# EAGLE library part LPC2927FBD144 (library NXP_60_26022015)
Short The LPC2926/2927/2929 combine an ARM968E-S CPU core with two integrated TCM blocks operating at frequencies of up to 125 MHz, Full-speed USB 2.0 OTG and device controller, CAN and LIN, 56 kB SRAM, up to 768 kB flash memory, external memory interface, three 10-bit ADCs, and multiple serial and parallel interfaces in a single chip targeted at consumer, industrial and communication markets. To optimize system power consumption, the LPC2926/2927/2929 has a very flexible Clock Generation Unit (CGU) that provides dynamic clock gating and scaling. AAL Eindhoven MK
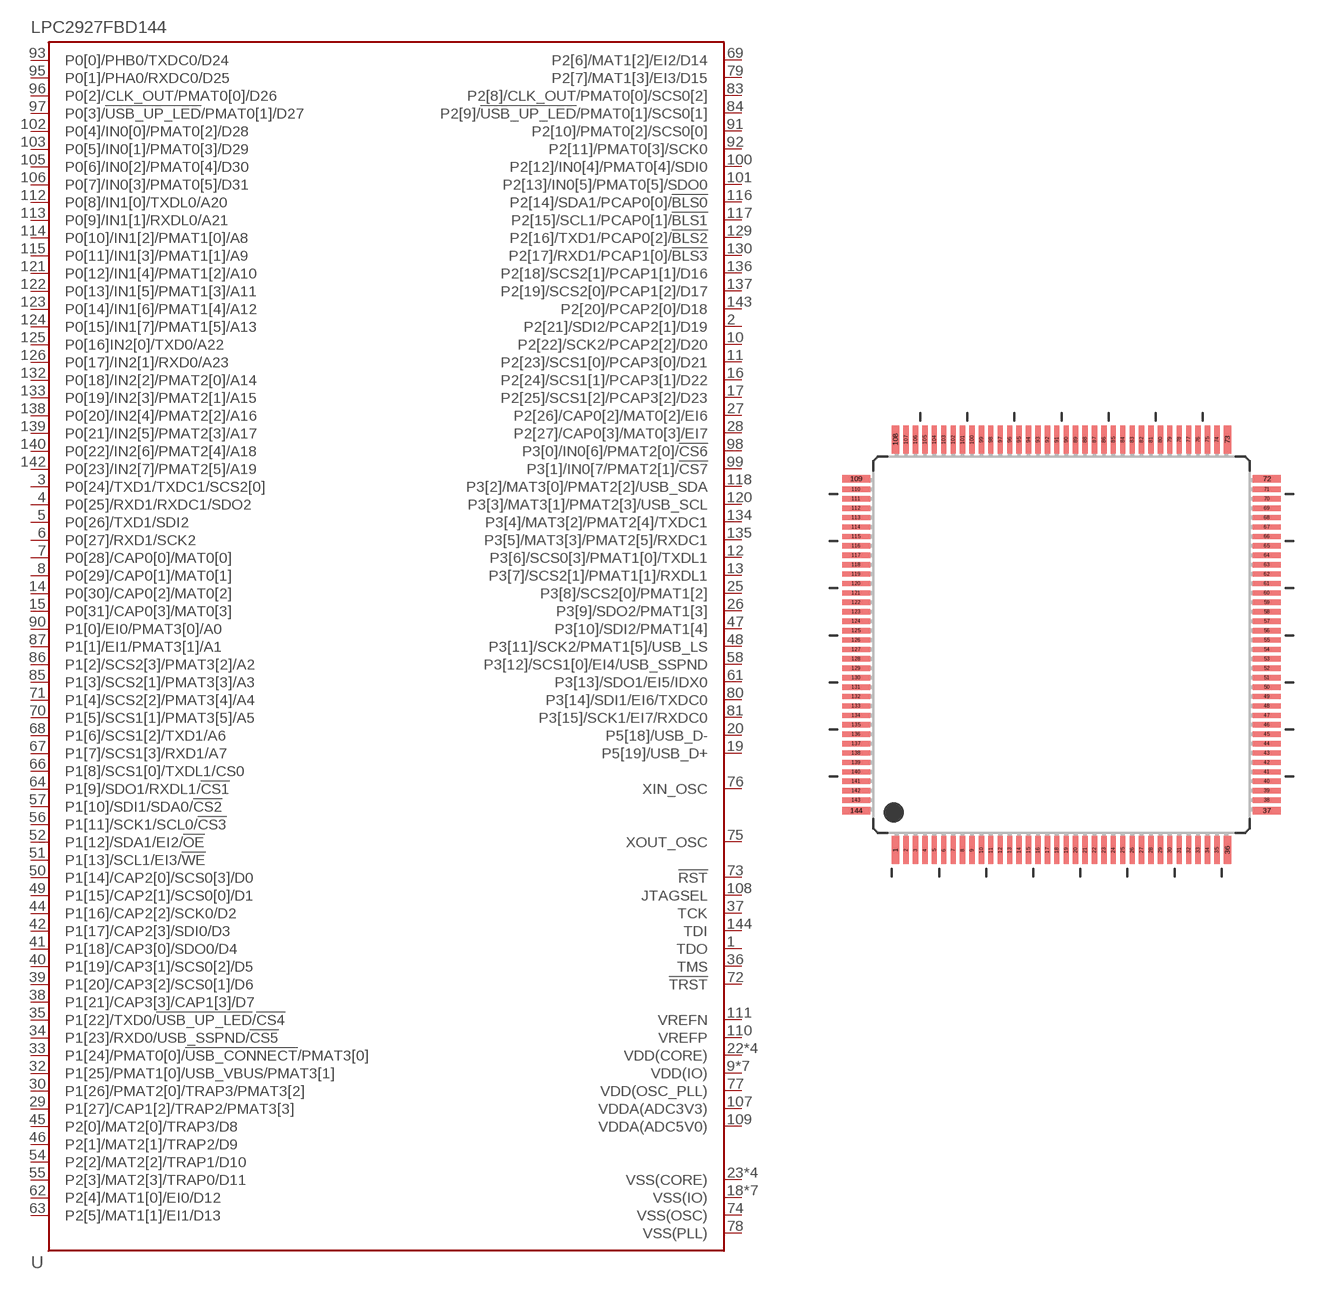
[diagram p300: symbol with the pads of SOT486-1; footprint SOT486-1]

Designator prefix U

## LPC2927FBD144 (FLASH: 512kB; SRAM: 56kB + 2 × 32kB TCM)  [SOT486-1]
1  TDO
2  P2[21]/SDI2/PCAP2[1]/D19
3  P0[24]/TXD1/TXDC1/SCS2[0]
4  P0[25]/RXD1/RXDC1/SDO2
5  P0[26]/TXD1/SDI2
6  P0[27]/RXD1/SCK2
7  P0[28]/CAP0[0]/MAT0[0]
8  P0[29]/CAP0[1]/MAT0[1]
9  VDD(IO)
10  P2[22]/SCK2/PCAP2[2]/D20
11  P2[23]/SCS1[0]/PCAP3[0]/D21
12  P3[6]/SCS0[3]/PMAT1[0]/TXDL1
13  P3[7]/SCS2[1]/PMAT1[1]/RXDL1
14  P0[30]/CAP0[2]/MAT0[2]
15  P0[31]/CAP0[3]/MAT0[3]
16  P2[24]/SCS1[1]/PCAP3[1]/D22
17  P2[25]/SCS1[2]/PCAP3[2]/D23
18  VSS(IO)
19  P5[19]/USB_D+
20  P5[18]/USB_D-
21  VDD(IO)
22  VDD(CORE)
23  VSS(CORE)
24  VSS(IO)
25  P3[8]/SCS2[0]/PMAT1[2]
26  P3[9]/SDO2/PMAT1[3]
27  P2[26]/CAP0[2]/MAT0[2]/EI6
28  P2[27]/CAP0[3]/MAT0[3]/EI7
29  P1[27]/CAP1[2]/TRAP2/PMAT3[3]
30  P1[26]/PMAT2[0]/TRAP3/PMAT3[2]
31  VDD(IO)
32  P1[25]/PMAT1[0]/USB_VBUS/PMAT3[1]
33  P1[24]/PMAT0[0]/!USB_CONNECT!/PMAT3[0]
34  P1[23]/RXD0/USB_SSPND/!CS5!
35  P1[22]/TXD0/!USB_UP_LED!/!CS4!
36  TMS
37  TCK
38  P1[21]/CAP3[3]/CAP1[3]/D7
39  P1[20]/CAP3[2]/SCS0[1]/D6
40  P1[19]/CAP3[1]/SCS0[2]/D5
41  P1[18]/CAP3[0]/SDO0/D4
42  P1[17]/CAP2[3]/SDI0/D3
43  VSS(IO)
44  P1[16]/CAP2[2]/SCK0/D2
45  P2[0]/MAT2[0]/TRAP3/D8
46  P2[1]/MAT2[1]/TRAP2/D9
47  P3[10]/SDI2/PMAT1[4]
48  P3[11]/SCK2/PMAT1[5]/USB_LS
49  P1[15]/CAP2[1]/SCS0[0]/D1
50  P1[14]/CAP2[0]/SCS0[3]/D0
51  P1[13]/SCL1/EI3/!WE!
52  P1[12]/SDA1/EI2/!OE!
53  VDD(IO)
54  P2[2]/MAT2[2]/TRAP1/D10
55  P2[3]/MAT2[3]/TRAP0/D11
56  P1[11]/SCK1/SCL0/!CS3!
57  P1[10]/SDI1/SDA0/!CS2!
58  P3[12]/SCS1[0]/EI4/USB_SSPND
59  VSS(CORE)
60  VDD(CORE)
61  P3[13]/SDO1/EI5/IDX0
62  P2[4]/MAT1[0]/EI0/D12
63  P2[5]/MAT1[1]/EI1/D13
64  P1[9]/SDO1/RXDL1/!CS1!
65  VSS(IO)
66  P1[8]/SCS1[0]/TXDL1/CS0
67  P1[7]/SCS1[3]/RXD1/A7
68  P1[6]/SCS1[2]/TXD1/A6
69  P2[6]/MAT1[2]/EI2/D14
70  P1[5]/SCS1[1]/PMAT3[5]/A5
71  P1[4]/SCS2[2]/PMAT3[4]/A4
72  !TRST!
73  !RST!
74  VSS(OSC)
75  XOUT_OSC
76  XIN_OSC
77  VDD(OSC_PLL)
78  VSS(PLL)
79  P2[7]/MAT1[3]/EI3/D15
80  P3[14]/SDI1/EI6/TXDC0
81  P3[15]/SCK1/EI7/RXDC0
82  VDD(IO)
83  P2[8]/CLK_OUT/PMAT0[0]/SCS0[2]
84  P2[9]/!USB_UP_LED!/PMAT0[1]/SCS0[1]
85  P1[3]/SCS2[1]/PMAT3[3]/A3
86  P1[2]/SCS2[3]/PMAT3[2]/A2
87  P1[1]/EI1/PMAT3[1]/A1
88  VSS(CORE)
89  VDD(CORE)
90  P1[0]/EI0/PMAT3[0]/A0
91  P2[10]/PMAT0[2]/SCS0[0]
92  P2[11]/PMAT0[3]/SCK0
93  P0[0]/PHB0/TXDC0/D24
94  VSS(IO)
95  P0[1]/PHA0/RXDC0/D25
96  P0[2]/CLK_OUT/PMAT0[0]/D26
97  P0[3]/!USB_UP_LED!/PMAT0[1]/D27
98  P3[0]/IN0[6]/PMAT2[0]/!CS6!
99  P3[1]/IN0[7/PMAT2[1]/!CS7!
100  P2[12]/IN0[4]/PMAT0[4]/SDI0
101  P2[13]/IN0[5]/PMAT0[5]/SDO0
102  P0[4]/IN0[0]/PMAT0[2]/D28
103  P0[5]/IN0[1]/PMAT0[3]/D29
104  VDD(IO)
105  P0[6]/IN0[2]/PMAT0[4]/D30
106  P0[7]/IN0[3]/PMAT0[5]/D31
107  VDDA(ADC3V3)
108  JTAGSEL
109  VDDA(ADC5V0)
110  VREFP
111  VREFN
112  P0[8]/IN1[0]/TXDL0/A20
113  P0[9]/IN1[1]/RXDL0/A21
114  P0[10]/IN1[2]/PMAT1[0]/A8
115  P0[11]/IN1[3]/PMAT1[1]/A9
116  P2[14]/SDA1/PCAP0[0]/!BLS0!
117  P2[15]/SCL1/PCAP0[1]/!BLS1!
118  P3[2]/MAT3[0]/PMAT2[2]/USB_SDA
119  VSS(IO)
120  P3[3]/MAT3[1]/PMAT2[3]/USB_SCL
121  P0[12]/IN1[4]/PMAT1[2]/A10
122  P0[13]/IN1[5]/PMAT1[3]/A11
123  P0[14]/IN1[6]/PMAT1[4]/A12
124  P0[15]/IN1[7]/PMAT1[5]/A13
125  P0[16]IN2[0]/TXD0/A22
126  P0[17]/IN2[1]/RXD0/A23
127  VDD(CORE)
128  VSS(CORE)
129  P2[16]/TXD1/PCAP0[2]/!BLS2!
130  P2[17]/RXD1/PCAP1[0]/!BLS3!
131  VDD(IO)
132  P0[18]/IN2[2]/PMAT2[0]/A14
133  P0[19]/IN2[3]/PMAT2[1]/A15
134  P3[4]/MAT3[2]/PMAT2[4]/TXDC1
135  P3[5]/MAT3[3]/PMAT2[5]/RXDC1
136  P2[18]/SCS2[1]/PCAP1[1]/D16
137  P2[19]/SCS2[0]/PCAP1[2]/D17
138  P0[20]/IN2[4]/PMAT2[2]/A16
139  P0[21]/IN2[5]/PMAT2[3]/A17
140  P0[22]/IN2[6]/PMAT2[4]/A18
141  VSS(IO)
142  P0[23]/IN2[7]/PMAT2[5]/A19
143  P2[20]/PCAP2[0]/D18
144  TDI

## Footprint SOT486-1 (pad centres in mm)
SOT486-1 LQFP144: plastic low profile quad flat package; 144 leads; body 20 x 20 x 1.4 mm JEDEC: MS-026 IEC: 136E23
smd 0.4 x 1.5: 1 -8.81,-10.9; 36 8.81,-10.9; 73 8.81,10.9; 108 -8.81,10.9
smd 0.28 x 1.5: 2 -8.25,-10.9; 3 -7.75,-10.9; 4 -7.25,-10.9; 5 -6.75,-10.9; 6 -6.25,-10.9; 7 -5.75,-10.9; 8 -5.25,-10.9; 9 -4.75,-10.9; 10 -4.25,-10.9; 11 -3.75,-10.9; 12 -3.25,-10.9; 13 -2.75,-10.9; 14 -2.25,-10.9; 15 -1.75,-10.9; 16 -1.25,-10.9; 17 -0.75,-10.9; 18 -0.25,-10.9; 19 0.25,-10.9; 20 0.75,-10.9; 21 1.25,-10.9; 22 1.75,-10.9; 23 2.25,-10.9; 24 2.75,-10.9; 25 3.25,-10.9; 26 3.75,-10.9; 27 4.25,-10.9; 28 4.75,-10.9; 29 5.25,-10.9; 30 5.75,-10.9; 31 6.25,-10.9; 32 6.75,-10.9; 33 7.25,-10.9; 34 7.75,-10.9; 35 8.25,-10.9; 74 8.25,10.9; 75 7.75,10.9; 76 7.25,10.9; 77 6.75,10.9; 78 6.25,10.9; 79 5.75,10.9; 80 5.25,10.9; 81 4.75,10.9; 82 4.25,10.9; 83 3.75,10.9; 84 3.25,10.9; 85 2.75,10.9; 86 2.25,10.9; 87 1.75,10.9; 88 1.25,10.9; 89 0.75,10.9; 90 0.25,10.9; 91 -0.25,10.9; 92 -0.75,10.9; 93 -1.25,10.9; 94 -1.75,10.9; 95 -2.25,10.9; 96 -2.75,10.9; 97 -3.25,10.9; 98 -3.75,10.9; 99 -4.25,10.9; 100 -4.75,10.9; 101 -5.25,10.9; 102 -5.75,10.9; 103 -6.25,10.9; 104 -6.75,10.9; 105 -7.25,10.9; 106 -7.75,10.9; 107 -8.25,10.9
smd 1.5 x 0.4: 37 10.9,-8.81; 72 10.9,8.81; 109 -10.9,8.81; 144 -10.9,-8.81
smd 1.5 x 0.28: 38 10.9,-8.25; 39 10.9,-7.75; 40 10.9,-7.25; 41 10.9,-6.75; 42 10.9,-6.25; 43 10.9,-5.75; 44 10.9,-5.25; 45 10.9,-4.75; 46 10.9,-4.25; 47 10.9,-3.75; 48 10.9,-3.25; 49 10.9,-2.75; 50 10.9,-2.25; 51 10.9,-1.75; 52 10.9,-1.25; 53 10.9,-0.75; 54 10.9,-0.25; 55 10.9,0.25; 56 10.9,0.75; 57 10.9,1.25; 58 10.9,1.75; 59 10.9,2.25; 60 10.9,2.75; 61 10.9,3.25; 62 10.9,3.75; 63 10.9,4.25; 64 10.9,4.75; 65 10.9,5.25; 66 10.9,5.75; 67 10.9,6.25; 68 10.9,6.75; 69 10.9,7.25; 70 10.9,7.75; 71 10.9,8.25; 110 -10.9,8.25; 111 -10.9,7.75; 112 -10.9,7.25; 113 -10.9,6.75; 114 -10.9,6.25; 115 -10.9,5.75; 116 -10.9,5.25; 117 -10.9,4.75; 118 -10.9,4.25; 119 -10.9,3.75; 120 -10.9,3.25; 121 -10.9,2.75; 122 -10.9,2.25; 123 -10.9,1.75; 124 -10.9,1.25; 125 -10.9,0.75; 126 -10.9,0.25; 127 -10.9,-0.25; 128 -10.9,-0.75; 129 -10.9,-1.25; 130 -10.9,-1.75; 131 -10.9,-2.25; 132 -10.9,-2.75; 133 -10.9,-3.25; 134 -10.9,-3.75; 135 -10.9,-4.25; 136 -10.9,-4.75; 137 -10.9,-5.25; 138 -10.9,-5.75; 139 -10.9,-6.25; 140 -10.9,-6.75; 141 -10.9,-7.25; 142 -10.9,-7.75; 143 -10.9,-8.25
